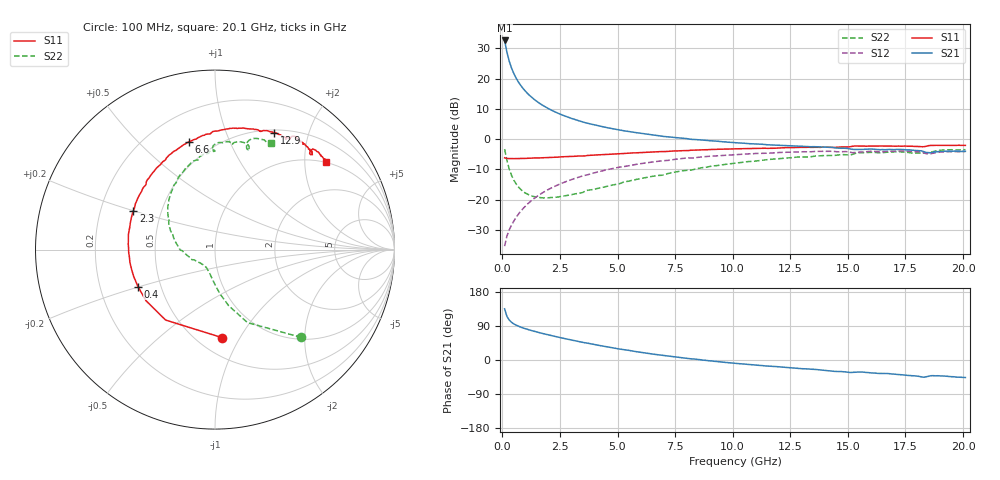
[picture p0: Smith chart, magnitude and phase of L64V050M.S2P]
!  Infineon Technologies AG
! BFR380L3 , PF131585-7, No.6, Th 09.10.01, soldered on pcb-board, measured with PP GSG850
!  Vce=4.0 V,  Ic=50.0 mA
! Common Emitter S-Parameters:  15. November 2001
#  GHz  S  MA  R  50
! f  S11  S21  S12  S22
! GHz  Mag  Ang  Mag  Ang  Mag  Ang  Mag  Ang
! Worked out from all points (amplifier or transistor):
!   201 points, 100 MHz to 20.1 GHz, reference 50 ohm
!   highest |S21| = 32.6 dB at 100 MHz (marker M1)
!   |S21| within 3 dB of that: start of sweep to 177.2 MHz
!   unconditionally stable (mu >= 1): 957 MHz to 4.225 GHz
!   at 3.4 GHz: K = 1.02, MAG = 8.3 dB, |S12| = -12.4 dB
!   at 10.1 GHz: K = 0.95, MSG = 2.0 dB, |S12| = -5.1 dB
!   at 20.1 GHz: K = 0.99, MSG = 0.0 dB, |S12| = -4.1 dB
!   S11 on the Smith chart (normalised r, x): 100 MHz: 0.65, -0.84; 400 MHz: 0.37, -0.20; 2.3 GHz: 0.35, +0.20; 6.6 GHz: 0.37, +0.72; 12.9 GHz: 0.53, +1.50; 20.1 GHz: 0.97, +2.55
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0.1  0.492 -85.4  42.87 135.1  0.01703 62.8  0.6862 -45.5
0.2  0.4794 -125.1  27.4 115.0  0.02501 57.6  0.4449 -66.0
0.3  0.4783 -143.5  19.5 105.4  0.03171 59.4  0.322 -76.2
0.4  0.4762 -154.3  15.01 99.5  0.03799 62.1  0.2529 -83.0
0.5  0.477 -161.7  12.17 95.3  0.04426 64.2  0.2104 -88.0
0.6  0.4777 -167.0  10.21 92.0  0.05099 65.8  0.1822 -92.0
0.7  0.4793 -171.4  8.803 89.2  0.05764 67.0  0.1622 -95.7
0.8  0.4787 -175.0  7.738 86.8  0.06449 67.8  0.1477 -99.0
1  0.4815 179.2  6.232 82.6  0.07816 68.7  0.1287 -105.0
1.2  0.4853 174.2  5.222 78.9  0.09202 68.7  0.118 -110.4
1.5  0.4898 168.0  4.213 73.9  0.1128 68.4  0.1096 -117.7
1.8  0.4948 162.6  3.539 69.2  0.1338 67.4  0.1068 -124.5
2.3  0.5039 154.4  2.813 62.0  0.1679 64.9  0.1095 -135.4
3.5  0.5277 137.4  1.922 46.4  0.2479 57.4  0.1319 -154.5
5  0.5701 119.7  1.439 29.8  0.34 47.0  0.1811 -177.5
6.6  0.6173 103.8  1.166 15.0  0.4237 35.8  0.2463 161.7
6.8  0.6211 101.9  1.139 13.4  0.4338 34.3  0.252 159.3
10.1  0.6925 77.7  0.8745 -8.6  0.5555 12.5  0.4014 127.5
12.9  0.7313 63.1  0.7695 -22.4  0.6194 -5.1  0.5083 103.6
13.5  0.7342 60.3  0.7523 -24.6  0.6234 -8.3  0.5196 99.9
16.8  0.7702 48.0  0.6771 -36.1  0.6308 -24.4  0.6119 78.6
20.1  0.7905 38.4  0.6311 -46.2  0.6243 -38.3  0.6703 62.2
